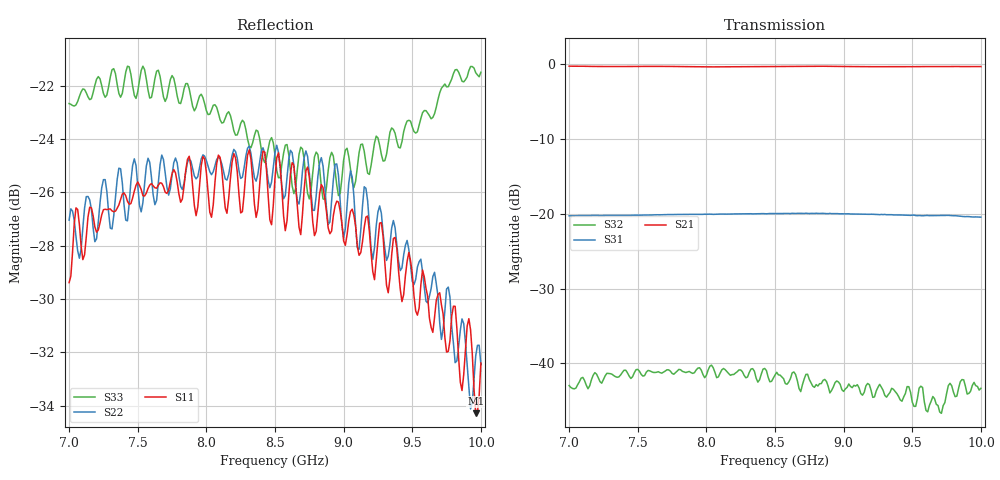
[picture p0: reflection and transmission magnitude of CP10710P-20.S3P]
! Amtery
! Email: info@amtery.com
! Phone: 886-2-2883-7839
! Model Number: CP10710P-20
! 3-port S-parameter measurement data for High Power Directional Coupler
! Frequency Range: 7 GHz to 10 GHz
! Port 1: Input
! Port 2: Output
! Port 3: Coupled
# Hz S dB R 50
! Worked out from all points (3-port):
!   241 points, 7 GHz to 10 GHz, reference 50 ohm
!   strongest paths, dB at 7 GHz, 7.75 GHz, 8.5 GHz, 9.25 GHz, 10 GHz:
!     S21: -0.2, -0.3, -0.3, -0.3, -0.3
!     S31: -20.3, -20.1, -20.0, -20.1, -20.4
!     S32: -43.0, -41.3, -41.6, -43.2, -43.3
!   lowest |S11| = -34.3 dB at 9.963 GHz (marker M1), VSWR 1.04, Z = 49.3 + j1.79 ohm
!   |S11| at or under -10 dB: start of sweep to end of sweep
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7e9  -29.38 -93.4  -0.25 -163.8  -20.28 -107.5
     -0.24 -164.0  -27.04 -80.4  -43.05 -23.0
     -20.26 -108.0  -42.97 -25.6  -22.67 -141.0
7.6375e9  -25.84 -131.1  -0.25 148.2  -20.13 -158.2
          -0.26 148.3  -26.30 -127.3  -41.47 -106.7
          -20.12 -158.6  -41.18 -107.4  -21.45 151.6
8.0875e9  -24.60 -159.3  -0.33 114.6  -20.06 166.1
          -0.33 114.8  -24.68 -166.3  -41.54 -154.6
          -20.03 165.4  -41.80 -155.9  -23.03 112.6
8.5e9  -25.46 174.2  -0.32 83.9  -19.99 133.0
       -0.28 84.2  -24.51 156.3  -41.92 162.7
       -19.95 132.4  -41.56 163.4  -24.60 84.8
9.2875e9  -27.65 143.4  -0.33 24.7  -20.12 68.9
          -0.32 25.1  -27.52 83.6  -43.95 96.1
          -20.09 68.8  -43.60 90.3  -24.82 40.0
9.7125e9  -30.21 130.7  -0.30 -7.1  -20.21 35.1
          -0.29 -6.7  -31.51 40.3  -45.59 81.4
          -20.20 34.9  -46.67 79.1  -22.09 6.5
9.775e9  -31.55 108.3  -0.31 -11.8  -20.22 29.6
         -0.29 -11.4  -29.94 31.1  -43.52 78.5
         -20.21 29.2  -42.66 76.3  -21.88 -3.8
9.9125e9  -30.74 115.7  -0.29 -22.2  -20.38 18.2
          -0.28 -21.8  -33.29 24.9  -43.43 60.8
          -20.36 18.0  -44.01 62.4  -21.43 -20.9
9.9625e9  -34.29 109.7  -0.30 -25.9  -20.42 14.4
          -0.30 -25.6  -32.13 6.6  -42.97 56.9
          -20.40 14.0  -42.98 55.2  -21.51 -23.1
1e10  -32.40 99.0  -0.29 -28.8  -20.44 11.4
      -0.29 -28.4  -32.46 19.0  -42.97 54.3
      -20.44 11.1  -43.33 52.9  -21.49 -29.6
